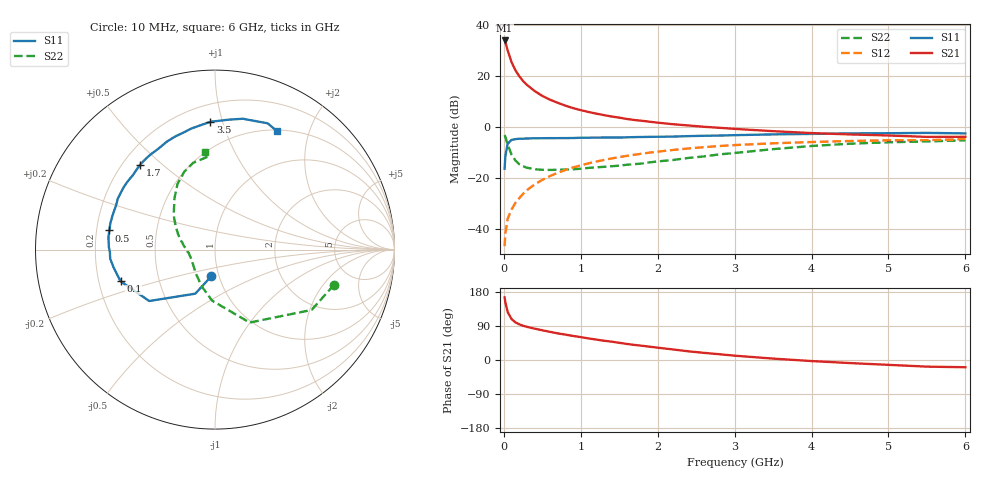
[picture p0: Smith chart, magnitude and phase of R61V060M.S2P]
! SIEMENS Small Signal Semiconductors
! BFR193
! Si NPN RF Bipolar Junction Transistor in SOT23
! VCE = 1 V  IC = 60 mA
! Common Emitter S-Parameters:  May  1996
# GHz  S  MA  R  50
!  f  S11  S21  S12  S22
! GHz  MAG  ANG  MAG  ANG  MAG  ANG  MAG  ANG
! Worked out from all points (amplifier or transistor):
!   36 points, 10 MHz to 6 GHz, reference 50 ohm
!   highest |S21| = 34.0 dB at 10 MHz (marker M1)
!   |S21| within 3 dB of that: start of sweep to 41.62 MHz
!   unconditionally stable (mu >= 1): start of sweep to 12.58 MHz; 179.1 MHz to 2.921 GHz; 5 GHz to end of sweep
!   at 250 MHz: K = 1.06, MAG = 20.7 dB, |S12| = -26.3 dB
!   at 1.4 GHz: K = 1.07, MAG = 6.7 dB, |S12| = -12.4 dB
!   at 6 GHz: K = 1.01, MAG = -0.2 dB, |S12| = -4.8 dB
!   S11 on the Smith chart (normalised r, x): 10 MHz: 0.92, -0.28; 100 MHz: 0.29, -0.15; 500 MHz: 0.25, +0.08; 1.7 GHz: 0.27, +0.42; 3.5 GHz: 0.32, +0.91; 6 GHz: 0.52, +1.53
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0.01  0.1502 -97.9  50.21 165.2  0.0045 70.4  0.6916 -16.5
0.02  0.269 -114.1  46.41 152.1  0.0081 69.5  0.6346 -32.0
0.05  0.4653 -142.0  32.06 126.4  0.0156 63.3  0.45 -64.6
0.1  0.5548 -161.5  18.82 108.2  0.0236 64.9  0.285 -93.2
0.15  0.5737 -170.0  13.08 99.4  0.032 67.5  0.2183 -109.6
0.2  0.5861 -175.0  9.947 94.2  0.0395 69.9  0.1846 -121.2
0.25  0.5858 -178.7  7.98 90.4  0.0482 71.2  0.1679 -130.8
0.3  0.5915 178.6  6.709 87.5  0.0569 72.2  0.1576 -136.6
0.4  0.5977 173.3  5.079 82.7  0.0736 72.7  0.1468 -146.9
0.5  0.5986 169.7  4.077 78.4  0.0907 72.3  0.1429 -155.1
0.6  0.6012 165.9  3.429 74.3  0.1078 71.2  0.1424 -159.9
0.8  0.602 159.3  2.619 67.0  0.142 68.7  0.145 -167.7
0.9  0.6041 155.6  2.343 63.5  0.159 67.2  0.1465 -171.7
1.1  0.613 149.3  1.967 57.0  0.1916 64.2  0.156 -176.7
1.3  0.6172 143.1  1.707 50.9  0.2236 60.6  0.1637 177.6
1.7  0.6299 131.7  1.365 39.7  0.2836 53.6  0.1848 168.0
2.2  0.6447 119.2  1.129 27.8  0.3519 44.7  0.2234 157.2
2.6  0.6686 109.2  1.005 18.9  0.399 37.5  0.2623 147.4
3.5  0.7123 92.1  0.824 3.7  0.4756 22.2  0.3651 128.2
4.5  0.7454 78.0  0.711 -8.1  0.5281 8.1  0.4667 111.5
5.5  0.7623 67.4  0.636 -17.5  0.5471 -4.5  0.5168 95.2
6  0.7449 62.3  0.639 -19.1  0.5758 -8.5  0.5459 96.1
